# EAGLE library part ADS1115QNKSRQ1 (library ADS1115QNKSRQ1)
Analog to Digital Converters - ADC Automotive 16-bit, 860-SPS, 4-ch, delta-sigma ADC with PGA, oscillator, VREF, comparator and I2C Source: Datasheet
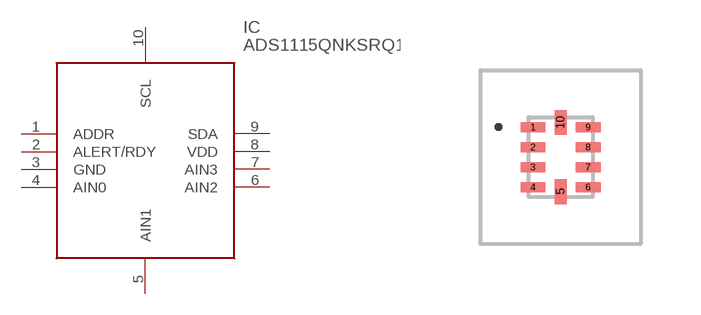
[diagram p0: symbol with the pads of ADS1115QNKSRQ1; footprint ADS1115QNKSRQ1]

Designator prefix IC

## ADS1115QNKSRQ1 (Description: Analog to Digital Converters - ADC Automotive 16-bit, 860-SPS, 4-ch, delta-sigma ADC with PGA, oscillator, VREF, comparator and I2C; Height: 0.6mm; Manufacturer_Name: Texas Instruments; Manufacturer_Part_Number: ADS1115QNKSRQ1; Mouser_Part_Number: 595-ADS1115QNKSRQ1; Mouser_Price-Stock: https://www.mouser.co.uk/ProductDetail/Texas-Instruments/ADS1115QNKSRQ1?qs=ulEaXIWI0c%252B%252BH1ufhGRAvg%3D%3D)  [ADS1115QNKSRQ1]
1  ADDR
2  ALERT/RDY
3  GND
4  AIN0
5  AIN1
6  AIN2
7  AIN3
8  VDD
9  SDA
10  SCL

## Footprint ADS1115QNKSRQ1 (pad centres in mm)
NKS0010A
smd 0.62 x 0.25: 1 -0.69,0.75; 2 -0.69,0.25; 3 -0.69,-0.25; 4 -0.69,-0.75; 6 0.69,-0.75; 7 0.69,-0.25; 8 0.69,0.25; 9 0.69,0.75
smd 0.3 x 0.62: 5 0,-0.865; 10 0,0.865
